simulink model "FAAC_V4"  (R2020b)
settings: Solver=VariableStepAuto  StartTime=0.0  StopTime=inf  MaxStep=0.2  RelTol=1e-3  EnableMultiTasking=on
libraries: fl_lib x11, sh_lib x6, nesl_utility x2, ee_lib x1

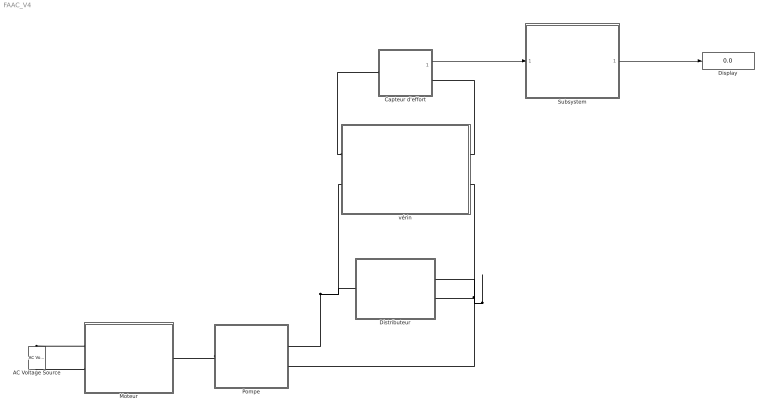
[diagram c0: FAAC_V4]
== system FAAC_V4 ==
  AC Voltage Source : fl_lib/Electrical/Electrical Sources/AC Voltage Source  amp=220 V  shift=64 deg  frequency=50 Hz  omega=0 rad/s
  Capteur d'effort : Subsystem
  Display : Display
  Distributeur : Subsystem
  Moteur : Subsystem
  Pompe : Subsystem
  Subsystem : Subsystem
  vérin : Subsystem
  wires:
  Capteur d'effort/1(output) -> Subsystem/1(In1)
  Subsystem/1(Out1) -> Display/1
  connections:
  Pompe/RConn2 -- Distributeur/RConn2 -- Distributeur/RConn1 -- vérin/LConn2
  Moteur/LConn1 -- AC Voltage Source/LConn1
  AC Voltage Source/RConn1 -- Moteur/LConn2
  Pompe/LConn1 -- Moteur/RConn1
  Pompe/RConn1 -- vérin/RConn2 -- Distributeur/LConn1
  vérin/RConn1 -- Capteur d'effort/LConn1
  vérin/LConn1 -- Capteur d'effort/RConn1

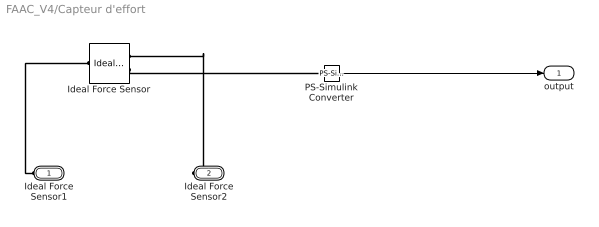
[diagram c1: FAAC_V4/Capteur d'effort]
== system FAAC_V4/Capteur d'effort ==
  Ideal Force Sensor : fl_lib/Mechanical/Mechanical Sensors/Ideal Force Sensor
  PS-Simulink Converter : nesl_utility/PS-Simulink Converter  PhysicalDomain=network_engine_domain  SubClassName=ps_output  LeftPortType=input  RightPortType=output  PseudoPeriodic=off  Frequencies=[]  Unit=N  AffineConversion=off
  Ideal Force Sensor1 : PMIOPort  Side=Left
  Ideal Force Sensor2 : PMIOPort  Port=2  Side=Right
  output : Outport
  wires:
  PS-Simulink Converter/1 -> output/1
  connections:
  Ideal Force Sensor/RConn2 -- PS-Simulink Converter/LConn1
  Ideal Force Sensor1/RConn1 -- Ideal Force Sensor/LConn1
  Ideal Force Sensor2/RConn1 -- Ideal Force Sensor/RConn1

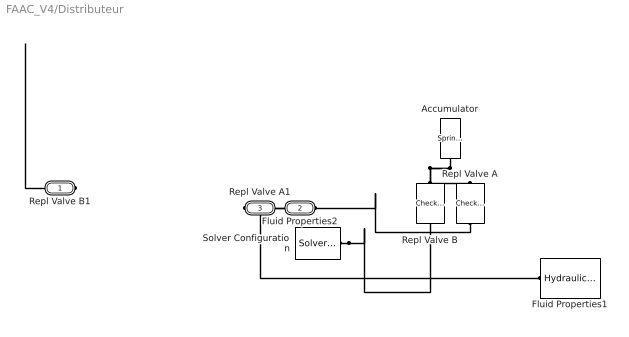
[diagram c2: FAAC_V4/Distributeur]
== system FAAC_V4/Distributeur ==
  Accumulator : sh_lib/Accumulators/Spring-Loaded Accumulator  capacity=15 l  pr_preload=0.5 Pa  pr_max=0.54e5 Pa  stiff_coeff=1e10 Pa/m^3  penetr_coeff=1e10 s*Pa/m^6  flow_rate_specify=off  flow_rate_priority=None  flow_rate=0.005 m^3/s  flow_rate_nominal_specify=off  flow_rate_nominal_unit=m^3/s  flow_rate_nominal_value=1  fluid_volume_specify=on  fluid_volume_priority=High  fluid_volume=5.6 l  fluid_volume_nominal_specify=off  fluid_volume_nominal_unit=m^3  fluid_volume_nominal_value=1  fluid_pressure_specify=off  fluid_pressure_priority=None  fluid_pressure=1.01325e+5 Pa  fluid_pressure_nominal_specify=off  fluid_pressure_nominal_unit=Pa  fluid_pressure_nominal_value=1
  Fluid Properties1 : sh_lib/Hydraulic Utilities/Hydraulic Fluid  Tag=Factory Generic  DataSource=1  SelFluid=9  SysTemp=60  TrapAir=0.005  ViscDerFactor=1  range_error=2
  Repl Valve A : sh_lib/Valves/Directional Valves/Check Valve  Tag=Factory Generic  area_max=1e-04 m^2  pres_crack=0.3e+04 Pa  pres_max=0.3e+05 Pa  C_d=0.7  A_leak=1e-12 m^2  lam_spec=1  B_lam=0.999  Re_cr=12  dynamic=0  tau=0.1 s  area_init=1e-12 m^2
  Repl Valve B : sh_lib/Valves/Directional Valves/Check Valve  Tag=Factory Generic  area_max=1e-04 m^2  pres_crack=0.03e+05 Pa  pres_max=0.4e+05 Pa  C_d=0.7  A_leak=1e-12 m^2  lam_spec=1  B_lam=0.999  Re_cr=12  dynamic=0  tau=0.1 s  area_init=1e-12 m^2
  Solver Configuration : nesl_utility/Solver Configuration  PhysicalDomain=network_engine_domain  SubClassName=solver  LeftPortType=input  RightPortType=generic  Tones=[]  Harmonics=[]  SimulateNoise=off  Profile=off  UseLocalSampling=off  EnableSwitchedLinearOptims=on  FrequencyDomain=off  UseCCode=off  RelTol=0.001  AbsTol=1e-06  MinStep=1e-09  ToWorkspace=off  RevertToSquareIcSolve=off  NumHomotopyIterations=100  PhasorMode=off  PhasorModeNumHarmonics=1  DoDC=off  ResidualTolerance=1e-9  UseLocalSolver=off  LocalSolverChoice=NE_BACKWARD_EULER_ADVANCER  LocalSolverSampleTime=.001  DoFixedCost=off  MaxNonlinIter=3  MaxModeIter=2  ComputeImpulses=off  ImpulseIterations=2  LinearAlgebra=auto  EquationFormulation=NE_TIME_EF  DelaysMemoryBudget=1024  AutomaticFiltering=on  FilteringTimeConstant=0.001  PartitionStorageMethod=AS_NEEDED  PartitionMemoryBudget=1024  PartitionMethod=FAST
  Repl Valve B1 : PMIOPort  Side=Left
  Fluid Properties2 : PMIOPort  Port=2  Side=Right
  Repl Valve A1 : PMIOPort  Port=3  Side=Right
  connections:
  Solver Configuration/RConn1 -- Repl Valve B/RConn1 -- Repl Valve B1/RConn1
  Repl Valve B/LConn1 -- Accumulator/RConn1 -- Repl Valve A/LConn1
  Fluid Properties1/RConn1 -- Fluid Properties2/RConn1
  Repl Valve A/RConn1 -- Repl Valve A1/RConn1

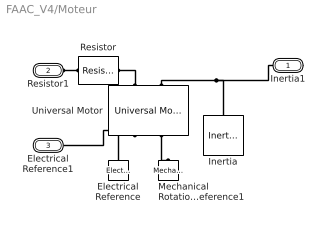
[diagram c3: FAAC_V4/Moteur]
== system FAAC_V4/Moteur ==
  Electrical Reference : fl_lib/Electrical/Electrical Elements/Electrical Reference
  Inertia : fl_lib/Mechanical/Rotational Elements/Inertia  inertia=0.01 kg*m^2  num_ports=foundation.enum.numPorts2.one  w_specify=off  w_priority=High  w=0 rad/s  w_nominal_specify=off  w_nominal_unit=rad/s  w_nominal_value=1  t_specify=off  t_priority=None  t=0 N*m  t_nominal_specify=off  t_nominal_unit=N*m  t_nominal_value=1
  Mechanical Rotational Reference1 : fl_lib/Mechanical/Rotational Elements/Mechanical Rotational Reference
  Resistor : fl_lib/Electrical/Electrical Elements/Resistor  R=9650 Ohm  i_specify=off  i_priority=None  i=0 A  i_nominal_specify=off  i_nominal_unit=A  i_nominal_value=1  v_specify=off  v_priority=None  v=0 V  v_nominal_specify=off  v_nominal_unit=V  v_nominal_value=1
  Universal Motor : ee_lib/Electromechanical/Brushed Motors/Universal Motor  parameterization=4  Ra=132.8 Ohm  Laf=0.1722 s*V/rad/A  w_rated=10 rpm  P_rated=140 W  V_dc=200 V  T_max=0.39 N*m  P_in=10 W  V_ac=10 V  I_ac=10 A  w_ac=10 Hz  Ltot=0.525 H  J=2e-4 kg*m^2  lam=1e-6 N*m/(rad/s)  speed0=0 rpm  resistance_ratio=1  alpha=[.00393, .00393] 1/K  Tmeas=25 degC  thermal_masses=[100, 100] J/K  initial_temperatures=[25, 25] degC
  Inertia1 : PMIOPort  Side=Right
  Resistor1 : PMIOPort  Port=2  Side=Left
  Electrical Reference1 : PMIOPort  Port=3  Side=Left
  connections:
  Universal Motor/LConn2 -- Inertia1/RConn1 -- Inertia/LConn1
  Universal Motor/RConn1 -- Electrical Reference1/RConn1 -- Electrical Reference/LConn1
  Universal Motor/LConn1 -- Resistor/RConn1
  Universal Motor/RConn2 -- Mechanical Rotational Reference1/LConn1
  Resistor/LConn1 -- Resistor1/RConn1

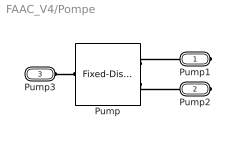
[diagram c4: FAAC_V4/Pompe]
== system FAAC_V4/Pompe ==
  Pump : sh_lib/Pumps and Motors/Fixed-Displacement Pump  Tag=Factory Generic  D=10 l/rev  loss_spec=1  w_nominal=10 rpm  pr_nominal=10 Pa  visc_nominal=18 cSt  dens_nominal=900 kg/m^3  efficiency_vol=0.92  no_load_torque=0 N*m  torque_pressure_coeff=1*(1.14e-06)*((0.92)/(0.8)-1 ) N*m/Pa  p_diff_eff_TLU=[100000.0, 1000000.0, 2000000.0] Pa  omega_eff_TLU=[25.0, 50.0, 100.0, 200.0, 300.0, 400.0] rad/s  vol_eff_TLU=[0.816, 0.908, 0.954, 0.977, 0.981, 0.984; 0.325, 0.663, 0.831, 0.916, 0.925, 0.946; 0.137, 0.568, 0.78, 0.892, 0.893, 0.91]  mech_eff_TLU=[0.996, 0.996, 0.996, 0.996, 0.996, 0.996; 0.988, 0.989, 0.989, 0.989, 0.989, 0.99; 0.981, 0.981, 0.982, 0.982, 0.983, 0.984]  p_diff_loss_TLU=[100000.0, 1000000.0, 2000000.0] Pa  omega_loss_TLU=[25.0, 50.0, 100.0, 200.0, 300.0, 400.0] rad/s  vol_loss_TLU=[0.023, 0.023, 0.023, 0.023, 0.0285, 0.032; 0.0844, 0.0842, 0.0845, 0.084, 0.1125, 0.108; 0.1079, 0.108, 0.11, 0.108, 0.1605, 0.18] * 1e-3 m^3/s  mech_loss_TLU=[0.002, 0.002, 0.002, 0.002, 0.002, 0.002; 0.0607, 0.0556, 0.0556, 0.0556, 0.0556, 0.0505; 0.1937, 0.1937, 0.1833, 0.1833, 0.1729, 0.1626] N*m  pressure_threshold=1e5 Pa  omega_threshold=10 rad/s  quadrant_check=0  pressure_check=0  min_valid_pressure=0 Pa  vol_eff_min=1e-3  vol_eff_max=1  mech_eff_min=1e-3  mech_eff_max=1
  Pump1 : PMIOPort  Side=Right
  Pump2 : PMIOPort  Port=2  Side=Right
  Pump3 : PMIOPort  Port=3  Side=Left
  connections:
  Pump/LConn1 -- Pump3/RConn1
  Pump/RConn1 -- Pump1/RConn1
  Pump/RConn2 -- Pump2/RConn1

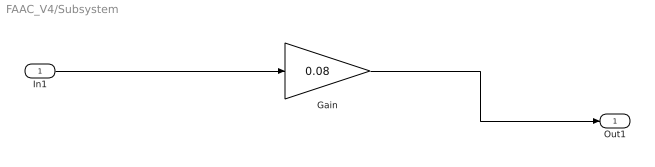
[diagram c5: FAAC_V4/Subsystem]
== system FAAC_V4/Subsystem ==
  In1 : Inport
  Gain : Gain  Gain=0.08
  Out1 : Outport
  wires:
  Gain/1 -> Out1/1
  In1/1 -> Gain/1

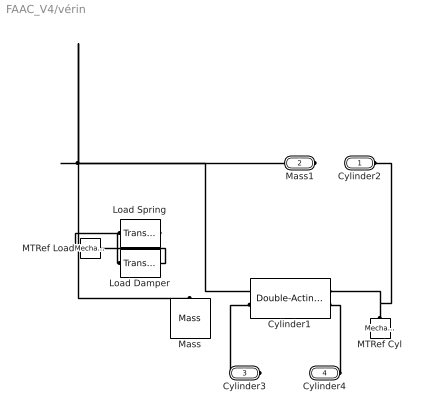
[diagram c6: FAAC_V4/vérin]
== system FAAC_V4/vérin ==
  Cylinder1 : sh_lib/Hydraulic Cylinders/Double-Acting Hydraulic Cylinder  Tag=Factory Generic  area_A=10 m^2  area_B=10 m^2  stroke=0.28 m  init_pos=0.14 m  dead_vol_A=5e-4 m^3  dead_vol_B=5e-4 m^3  init_pressure_A=0 Pa  init_pressure_B=0 Pa  k_sh=1.4  stiff=1e+07 N/m  D=150 N/(m/s)  hardstop_model=3  transition=0.1 mm  or=2
  Load Damper : fl_lib/Mechanical/Translational Elements/Translational Damper  Tag=Factory Generic  D=250 s*N/m  v_specify=off  v_priority=High  v=0 m/s  v_nominal_specify=off  v_nominal_unit=m/s  v_nominal_value=1  f_specify=off  f_priority=High  f=0 N  f_nominal_specify=off  f_nominal_unit=N  f_nominal_value=1
  Load Spring : fl_lib/Mechanical/Translational Elements/Translational Spring  Tag=Factory Generic  spr_rate=9.5e4 N/m  v_specify=off  v_priority=High  v=0 m/s  v_nominal_specify=off  v_nominal_unit=m/s  v_nominal_value=1  f_specify=off  f_priority=High  f=0 N  f_nominal_specify=off  f_nominal_unit=N  f_nominal_value=1  x_specify=on  x_priority=High  x=0.02 m  x_nominal_specify=off  x_nominal_unit=m  x_nominal_value=1
  MTRef Cyl : fl_lib/Mechanical/Translational Elements/Mechanical Translational Reference  Tag=Factory Generic
  MTRef Load : fl_lib/Mechanical/Translational Elements/Mechanical Translational Reference  Tag=Factory Generic
  Mass : fl_lib/Mechanical/Translational Elements/Mass  Tag=Factory Generic  mass=4.5 kg  num_ports=foundation.enum.numPorts2.one  v_specify=on  v_priority=High  v=0 m/s  v_nominal_specify=off  v_nominal_unit=m/s  v_nominal_value=1  f_specify=off  f_priority=High  f=0 N  f_nominal_specify=off  f_nominal_unit=N  f_nominal_value=1
  Cylinder2 : PMIOPort  Side=Left
  Mass1 : PMIOPort  Port=2  Side=Right
  Cylinder3 : PMIOPort  Port=3  Side=Right
  Cylinder4 : PMIOPort  Port=4  Side=Left
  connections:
  MTRef Load/LConn1 -- Load Damper/RConn1 -- Load Spring/RConn1
  MTRef Cyl/LConn1 -- Cylinder2/RConn1 -- Cylinder1/LConn1
  Load Spring/LConn1 -- Mass1/RConn1 -- Mass/LConn1 -- Cylinder1/RConn1 -- Load Damper/LConn1
  Cylinder1/LConn2 -- Cylinder4/RConn1
  Cylinder1/RConn2 -- Cylinder3/RConn1
